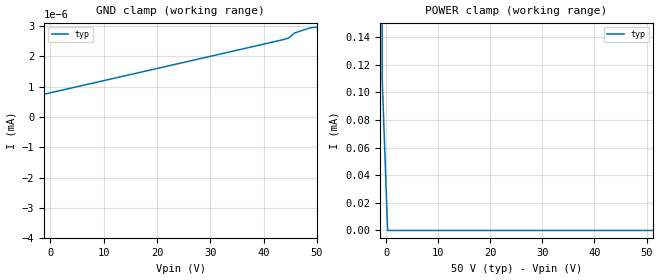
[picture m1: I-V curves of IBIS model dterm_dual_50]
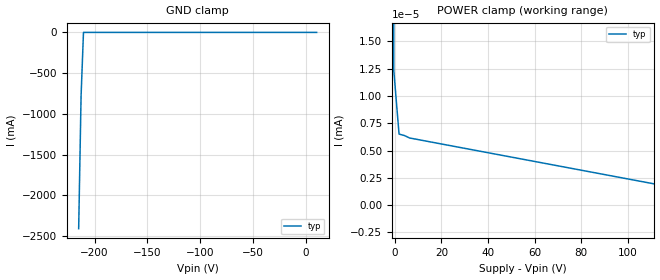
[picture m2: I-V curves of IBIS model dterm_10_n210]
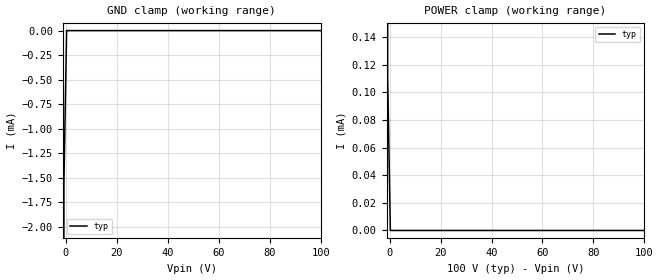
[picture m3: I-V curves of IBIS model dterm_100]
|Texas Instruments Incorporated
|tmux9612, 4 Data Lane 1:1 220V Switch
[IBIS Ver]   4.1
[File name]   tmux9612.ibs
[Date]   02/11/25
[File Rev]   1.0
[Source]
| Texas Instruments Incorporated.
| ASC-INT-MPD
| 12500 TI Blvd
| Dallas, TX - 75243
[Notes]   Revision History:
| Rev 1.0: 02/11/25
| - Initial version of the model
| - Model generated from simulations in SPECTRE
| - C_comp although listed in numerical order of value are
|   obtained from varying PVT conditions. For PVT conditions for
|   each specific value refer the buffer description under
|   respective [Model]. IBIS model user is responsible for using
|   appropriate C_comp to simulate for Signal Integrity.
[Disclaimer]
| This model is designed as an aid for customers of Texas Instruments.
| TI and its licensors and suppliers make no warranties, either expressed
| or implied, with respect to this  model, including the warranties of
| merchantability or fitness for a particular purpose. The model is
| provided solely on an "as is" basis. The entire risk as to its quality
| and performance is with the customer.
| This model is subject to change without notice. Texas Instruments
| Incorporated is not responsible for updating this model.
[Copyright]
(C) Copyright 2025 Texas Instruments Incorporated.All rights reserved.
|  Component TMUX9612RUM 16-pin - RUM package
|  Part # TMUX9612RUM
[Component]   TMUX9612RUM
[Manufacturer]  TI
[Package]
|   typ   min   max
R_pkg   0.0668   NA   NA
L_pkg   2.1992nH   NA   NA
C_pkg   0.2884pF   NA   NA
[Pin]   signal_name   model_name
   1   VSS   power
   2   SEL1   inbuf
   3   GND   gnd
   4   SEL4   inbuf
   5   D4   dterm
   6   S4   sterm
   7   S3   sterm
   8   D3   dterm
   9   VDD   power
   10   VOUT   nc
   11   SEL3   inbuf
   12   SEL2   inbuf
   13   D2   dterm
   14   S2   sterm
   15   S1   sterm
   16   D1   dterm
[Series Switch Groups]
On 1 /
On 2 /
On 3 /
On 4 /
Off 1 /
[Series Pin Mapping]  pin_2 model_name function_table_group
|  15  16   switch_dual_50   1
|  14  13   switch_dual_50   1
|  7   8   switch_dual_50   1
|  6   5   switch_dual_50   1
|  15  16   switch_10_n210   1
|  14  13   switch_10_n210   1
|   7   8   switch_10_n210   1
|   6   5   switch_10_n210   1
|  15  16   switch_100   1
|  14  13   switch_100   1
|   7   8   switch_100   1
|   6   5   switch_100   1
  15  16   switch_220   1
  14  13   switch_220   1
   7   8   switch_220   1
   6   5   switch_220   1
|  15  16  switch_dual_110   1
|  14  13  switch_dual_110   1
|   7   8  switch_dual_110   1
|   6   5  switch_dual_110   1
[Model Selector] dterm
dterm_dual_50 Use for operation at +/-50V
dterm_10_-210 Use for operation at 10V
dterm_100 Use for operation at 100V
dterm_220 Use for operation at 220V
dterm_dual_110 Use for operation at +/-110V
[Model Selector] sterm
sterm_dual_50 Use for operation at +/-50V
sterm_10_-210 Use for operation at 10V
sterm_100 Use for operation at 100V
sterm_220 Use for operation at 220V
sterm_dual_110 Use for operation at +/-110V
[Model Selector] inbuf
inbuf_dual_50 Use for operation at +/-50V
inbuf_10_-210 Use for operation at 10V
inbuf_100 Use for operation at 100V
inbuf_220 Use for operation at 220V
inbuf_dual_110 Use for operation at +/-110V
| switch_dual_50
[Model]   switch_dual_50
Model_type   Series_switch
|   typ   min   max
C_comp   6.362683e-12   NA   NA
[Voltage Range]   50   NA   NA
[Power Clamp Reference]   50   NA   NA
[Temperature Range]   27   NA   NA
[On]
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[Off]
|   typ   min   max
[R Series]   10G   NA   NA
| switch_10_n210
[Model]   switch_10_n210
Model_type   Series_switch
|   typ   min   max
C_comp   2.533030e-12   NA   NA
[Voltage Range]   10_210   NA   NA
[Power Clamp Reference]   10_210   NA   NA
[Temperature Range]   27   NA   NA
[On]
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[Off]
|   typ   min   max
[R Series]   10G   NA   NA
| switch_100
[Model]   switch_100
Model_type   Series_switch
|   typ   min   max
C_comp   1.008417e-11   NA   NA
[Voltage Range]   100   NA   NA
[Power Clamp Reference]   100   NA   NA
[Temperature Range]   27   NA   NA
[On]
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[Off]
|   typ   min   max
[R Series]   10G   NA   NA
| switch_220
[Model]   switch_220
Model_type   Series_switch
|   typ   min   max
C_comp   1.008417e-11   NA   NA
[Voltage Range]   220   NA   NA
[Power Clamp Reference]   220   NA   NA
[Temperature Range]   27   NA   NA
[On]
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[Off]
|   typ   min   max
[R Series]   10G   NA   NA
| switch_dual_110
[Model]   switch_dual_110
Model_type   Series_switch
|   typ   min   max
C_comp   6.362683e-12   NA   NA
[Voltage Range]   110   NA   NA
[Power Clamp Reference]   110   NA   NA
[Temperature Range]   27   NA   NA
[On]
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[Off]
|   typ   min   max
[R Series]   10G   NA   NA
| Models and submodels in the file (20): dterm_dual_50 (Terminator), dterm_10_n210 (Terminator), dterm_100 (Terminator), dterm_220 (Terminator), dterm_dual_110 (Terminator), switch_dual_50 (Series_switch), switch_10_n210 (Series_switch), switch_100 (Series_switch), switch_220 (Series_switch), switch_dual_110 (Series_switch), sterm_dual_50 (Terminator), sterm_10_n210 (Terminator), sterm_100 (Terminator), sterm_220 (Terminator), sterm_dual_110 (Terminator), inbuf_dual_50 (Input), inbuf_10_n210 (Input), inbuf_100 (Input), inbuf_220 (Input), inbuf_dual_110 (Input)
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| dterm_dual_50
[Model]   dterm_dual_50
Model_type   Terminator
|   typ   min   max
C_comp   6.362683e-12   NA   NA
[Voltage Range]   50   NA   NA
[Temperature Range]   27   NA   NA
[Power Clamp Reference]   50   NA   NA
[GND Clamp Reference]   0   NA   NA
[GND Clamp]
|   Voltage   I(typ)   I(min)   I(max)
-55V      -2.409A    NA         NA
-50.76V   -1.565mA   NA         NA
-49.7V    -1.2nA     NA         NA
43.64V    2.55nA     NA         NA
44.7V     2.605nA    NA         NA
45.76V    2.767nA    NA         NA
48.94V    2.949nA    NA         NA
50V       2.96nA     NA         NA
[POWER Clamp]
|   Voltage   I(typ)   I(min)   I(max)
-5V       1.055A     NA         NA
-1.818V   191.2mA    NA         NA
-757.6mV  111.3uA    NA         NA
303mV     2.957nA    NA         NA
100V      -1.212nA   NA         NA
| dterm_10_n210
[Model]   dterm_10_n210
Model_type   Terminator
|   typ   min   max
C_comp   2.533030e-12   NA   NA
[Voltage Range]   10_210   NA   NA
[Temperature Range]   27   NA   NA
[Power Clamp Reference]   10_210   NA   NA
[GND Clamp Reference]   0   NA   NA
[GND Clamp]
|   Voltage   I(typ)   I(min)   I(max)
-215V     -2.409A    NA         NA
-212.7V   -781.9mA   NA         NA
-210.5V   -102.8nA   NA         NA
10V       6.558nA    NA         NA
[POWER Clamp]
|   Voltage   I(typ)   I(min)   I(max)
-5V       1.055A     NA         NA
-2.727V   432.7mA    NA         NA
-454.5mV  12.37nA    NA         NA
1.818V    6.511nA    NA         NA
6.364V    6.153nA    NA         NA
220V      -2.413nA   NA         NA
| dterm_100
[Model]   dterm_100
Model_type   Terminator
|   typ   min   max
C_comp   1.008417e-11   NA   NA
[Voltage Range]   100   NA   NA
[Temperature Range]   27   NA   NA
[Power Clamp Reference]   100   NA   NA
[GND Clamp Reference]   0   NA   NA
[GND Clamp]
|   Voltage   I(typ)   I(min)   I(max)
-5V       -2.409A    NA         NA
-1.818V   -286.9mA   NA         NA
-757.6mV  -1.565mA   NA         NA
303mV     -1.198nA   NA         NA
100V      2.96nA     NA         NA
[POWER Clamp]
|   Voltage   I(typ)   I(min)   I(max)
-5V       1.055A     NA         NA
-1.818V   191.2mA    NA         NA
-758mV    111.3uA    NA         NA
303mV     2.957nA    NA         NA
100V      -1.21nA    NA         NA
